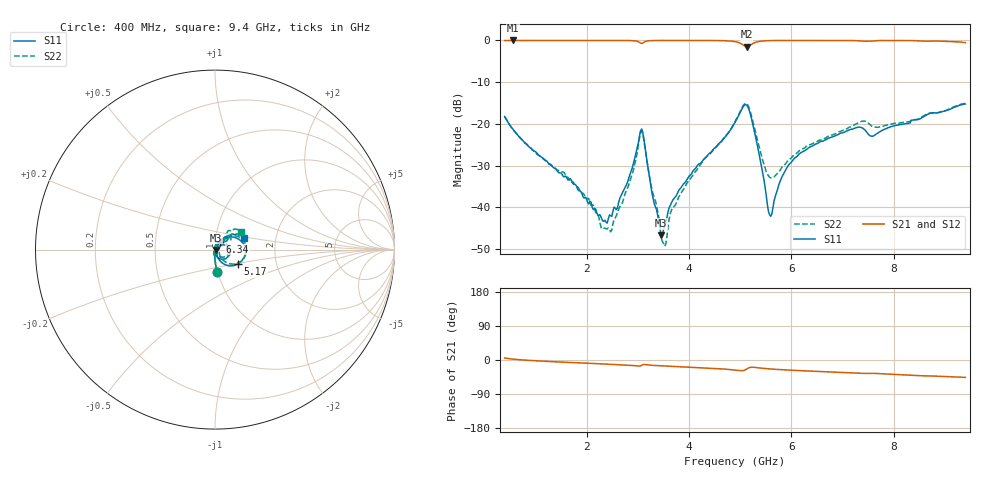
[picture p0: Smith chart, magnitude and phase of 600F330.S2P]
!  American Technical Ceramics  Date:  11/23/05
!  One Norden Lane
!  Huntington Station,  NY.  11746-2102
!  Tel:  (631) 622-4700  Fax:  (631) 622-4748
!  Part Number  600F330  Mounting Orientation: Horizontal
!  Description: Ultra Low ESR Microwave capacitors
!  Application: Coupling, Bypass, Tuning, DC Block
!  Filters, Matching
# GHZ S DB R 50
! Freq  |S11|  S11 Ph  |S21|  S21 Ph  |S12|  S12 Ph  |S22|  S22 Ph
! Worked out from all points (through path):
!   401 points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, 400 MHz to 9.4 GHz, reference 50 ohm
!   highest |S21| = 0.00 dB at 558 MHz (marker M1); lowest = -1.5 dB at 5.125 GHz (marker M2)
!   group delay of S21, straight-line fit = 14.1 ps
!   lowest |S11| = -46.7 dB at 3.46 GHz (marker M3), VSWR 1.01, Z = 50.4 - j0.148 ohm
!   |S11| at or under -10 dB: start of sweep to end of sweep
!   |S22| runs from -49.3 to -15.0 dB; largest |S21 - S12| = 0.0037
!   S11 on the Smith chart (normalised r, x): 400 MHz: 0.99, -0.25; 5.17 GHz: 1.27, -0.21; 6.34 GHz: 1.05, +0.09; 9.4 GHz: 1.37, +0.18
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0.4  -18.23 -84.8  -0.03 5.2  -0.04 5.1  -18.22 -84.7
0.558  -21.15 -87.0  0.00 2.4  -0.01 2.4  -21.16 -87.6
1.908  -36.56 -86.5  -0.01 -7.9  -0.01 -8.0  -36.55 -109.4
2.358  -43.05 -31.0  -0.01 -10.6  -0.01 -10.6  -44.95 -170.8
2.47  -41.95 -7.2  -0.01 -11.3  -0.01 -11.3  -45.82 147.9
2.808  -33.71 35.5  -0.02 -13.7  -0.02 -13.7  -35.18 92.6
3.078  -21.20 -20.4  -0.73 -13.9  -0.74 -14.0  -21.64 -6.3
3.415  -43.57 -47.0  0.00 -15.1  -0.01 -15.1  -42.49 -56.1
3.46  -46.68 -18.4  -0.01 -15.4  -0.01 -15.5  -47.39 -34.6
3.528  -44.45 20.5  -0.01 -15.9  0.00 -15.9  -49.27 8.6
3.663  -38.77 42.5  -0.01 -16.8  0.00 -16.9  -40.50 53.9
3.843  -35.31 52.3  -0.01 -17.9  -0.01 -18.0  -36.60 63.3
4.9  -19.62 41.8  -0.28 -26.6  -0.29 -26.6  -19.47 46.2
5.125  -15.46 -13.6  -1.51 -24.1  -1.51 -24.2  -15.12 -6.5
5.17  -16.44 -32.6  -1.35 -20.7  -1.36 -20.8  -16.01 -24.4
5.575  -41.72 -17.4  -0.05 -23.5  -0.05 -23.5  -32.73 -16.4
5.913  -30.51 60.9  -0.01 -26.3  -0.01 -26.4  -29.09 35.7
6.34  -25.69 58.8  -0.01 -29.1  -0.01 -29.1  -25.04 42.8
6.408  -25.30 59.1  -0.01 -29.5  -0.01 -29.5  -24.74 44.4
7.375  -20.89 41.2  -0.14 -35.4  -0.14 -35.4  -19.38 39.7
7.915  -20.78 51.4  0.00 -37.3  -0.01 -37.4  -20.17 40.5
9.4  -15.22 21.0  -0.52 -45.9  -0.53 -46.0  -15.03 33.7
